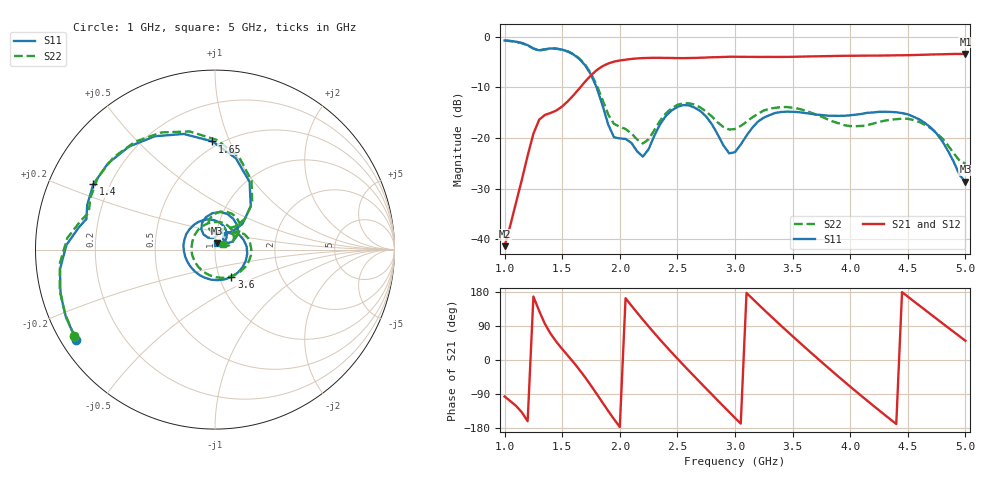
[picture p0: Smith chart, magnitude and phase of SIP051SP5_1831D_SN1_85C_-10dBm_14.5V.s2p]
# GHz  S  dB  R  50
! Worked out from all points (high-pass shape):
!   81 points, 1 GHz to 5 GHz, reference 50 ohm
!   highest |S21| = -3.35 dB at 5 GHz (marker M1); lowest = -41.4 dB at 1 GHz (marker M2)
!   |S21| within 3 dB of the highest: 1.814 GHz to end of sweep
!   lowest |S11| = -28.6 dB at 5 GHz (marker M3), VSWR 1.08, Z = 51.2 + j3.54 ohm
!   |S11| at or under -10 dB: 1.799 GHz to end of sweep
!   |S22| runs from -25.0 to -0.7 dB; largest |S21 - S12| = 0.0021
!   S11 on the Smith chart (normalised r, x): 1 GHz: 0.04, -0.30; 1.4 GHz: 0.14, +0.25; 1.65 GHz: 0.46, +0.87; 3.6 GHz: 1.14, -0.36; 5 GHz: 1.02, +0.07
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1  -0.71 -147.1  -41.37 -96.3  -41.24 -94.2  -0.72 -148.3
1.25  -2.29 170.7  -19.14 167.4  -19.13 167.5  -2.32 168.0
1.4  -2.27 151.7  -15.03 69.0  -15.03 69.0  -2.31 148.4
1.65  -4.39 91.3  -10.16 -26.0  -10.14 -26.0  -4.29 88.8
1.7  -5.65 77.1  -8.82 -46.1  -8.80 -46.1  -5.50 75.1
1.85  -13.53 43.0  -5.79 -112.4  -5.79 -112.5  -12.44 45.7
2  -20.07 74.8  -4.66 -176.9  -4.64 -176.9  -17.78 65.6
2.2  -23.67 101.4  -4.19 106.5  -4.19 106.6  -21.08 86.3
2.35  -17.26 123.8  -4.14 53.5  -4.13 53.6  -16.55 105.0
2.55  -13.48 82.5  -4.20 -12.5  -4.17 -12.5  -13.12 73.3
2.75  -15.75 38.5  -4.08 -75.6  -4.07 -75.5  -14.79 40.4
3  -22.78 50.5  -3.93 -152.8  -3.92 -152.9  -18.21 41.9
3.15  -17.96 50.1  -3.95 162.1  -3.95 162.2  -15.91 38.8
3.35  -15.04 6.0  -3.97 104.5  -3.96 104.5  -14.02 9.8
3.6  -15.02 -59.0  -3.89 35.4  -3.88 35.4  -14.53 -39.1
3.7  -15.35 -84.7  -3.85 8.4  -3.84 8.4  -15.33 -62.7
3.85  -15.60 -121.2  -3.78 -31.3  -3.77 -31.3  -16.72 -102.5
4.05  -15.37 -166.2  -3.73 -82.8  -3.72 -82.9  -17.66 -166.3
4.35  -14.83 130.8  -3.67 -156.9  -3.68 -157.0  -16.38 105.0
4.5  -15.31 100.3  -3.62 167.3  -3.61 167.4  -16.18 69.7
4.7  -17.95 61.8  -3.49 120.3  -3.48 120.4  -18.08 32.1
5  -28.64 69.1  -3.35 50.8  -3.35 50.7  -25.04 37.3
